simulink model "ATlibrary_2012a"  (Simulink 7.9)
settings: Solver=ode45  StartTime=0.0  StopTime=10.0  RelTol=1e-3
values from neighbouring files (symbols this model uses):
  params = []    [setParams.m]
  simopt = []    [setParams.m]
libraries: simulink x5, dspswit3 x1

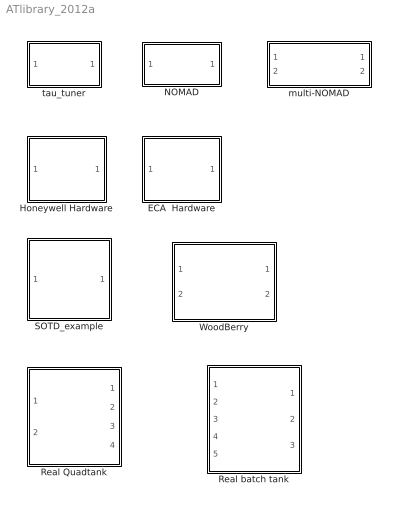
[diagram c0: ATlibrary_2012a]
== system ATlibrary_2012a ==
  ECA  Hardware : Subsystem
  Honeywell Hardware : Subsystem
  NOMAD : Subsystem  VariantObject=simopt.ID~=0
  Real Quadtank : Subsystem  AncestorBlock=tank/Real Quadtank  mask{h=0.01}
  Real batch tank : Subsystem  AncestorBlock=tank/Real Quadtank  mask{h=0.05}
  SOTD_example : Subsystem
  WoodBerry : Subsystem
  multi-NOMAD : Subsystem
  tau_tuner : Subsystem

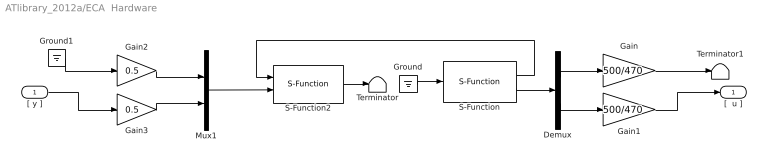
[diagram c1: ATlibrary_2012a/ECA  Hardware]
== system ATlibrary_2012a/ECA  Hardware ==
  "[ y ]" : Inport
  Demux : Demux  Outputs=2
  Gain : Gain  Gain=500/470
  Gain1 : Gain  Gain=500/470
  Gain2 : Gain  Gain=0.5
  Gain3 : Gain  Gain=0.5
  Ground : Ground
  Ground1 : Ground
  Mux1 : Mux  Inputs=2
  S-Function : S-Function  FunctionName=analogin  Parameters=simopt.h [1 0]  EnableBusSupport=off
  S-Function2 : S-Function  FunctionName=analogout  Parameters=simopt.h [1 0]  EnableBusSupport=off
  Terminator : Terminator
  Terminator1 : Terminator
  "[  u ]" : Outport  InitialOutput=0
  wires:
  Gain3/1 -> Mux1/2
  Gain2/1 -> Mux1/1
  Gain1/1 -> "[  u ]"/1
  Demux/2 -> Gain1/1
  Demux/1 -> Gain/1
  Gain/1 -> Terminator1/1
  Ground1/1 -> Gain2/1
  "[ y ]"/1 -> Gain3/1
  Mux1/1 -> S-Function2/2
  S-Function/2 -> Demux/1
  S-Function/1 -> S-Function2/1
  S-Function2/1 -> Terminator/1
  Ground/1 -> S-Function/1

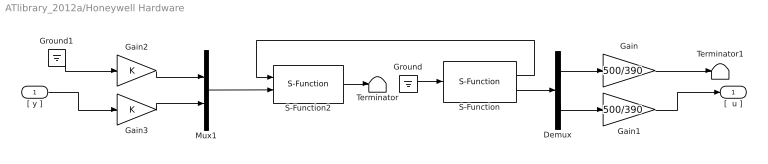
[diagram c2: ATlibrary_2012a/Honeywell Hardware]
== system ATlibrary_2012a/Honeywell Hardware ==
  "[ y ]" : Inport
  Demux : Demux  Outputs=2
  Gain : Gain  Gain=500/390
  Gain1 : Gain  Gain=500/390
  Gain2 : Gain
  Gain3 : Gain
  Ground : Ground
  Ground1 : Ground
  Mux1 : Mux  Inputs=2
  S-Function : S-Function  FunctionName=analogin  Parameters=simopt.h [1 0]  EnableBusSupport=off
  S-Function2 : S-Function  FunctionName=analogout  Parameters=simopt.h [1 0]  EnableBusSupport=off
  Terminator : Terminator
  Terminator1 : Terminator
  "[  u ]" : Outport  InitialOutput=0
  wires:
  Ground/1 -> S-Function/1
  S-Function2/1 -> Terminator/1
  S-Function/1 -> S-Function2/1
  S-Function/2 -> Demux/1
  Mux1/1 -> S-Function2/2
  "[ y ]"/1 -> Gain3/1
  Ground1/1 -> Gain2/1
  Gain/1 -> Terminator1/1
  Demux/1 -> Gain/1
  Demux/2 -> Gain1/1
  Gain1/1 -> "[  u ]"/1
  Gain2/1 -> Mux1/1
  Gain3/1 -> Mux1/2

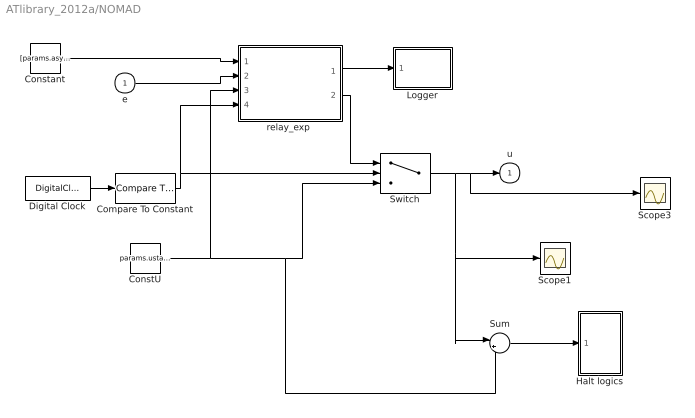
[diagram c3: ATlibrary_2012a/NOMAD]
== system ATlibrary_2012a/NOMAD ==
  e : Inport
  Compare To Constant : simulink/Logic and Bit Operations/Compare To Constant  relop=>=  const=params.expStartTime  OutDataTypeStr=boolean
  ConstU : Constant  Value=params.ustart  SampleTime=simopt.h
  Constant : Constant  Value=[params.asym simopt.h 1 simopt.uon params.hyst params.noiseMeasureTime]
  Digital Clock : DigitalClock  SampleTime=simopt.h
  Halt logics : Subsystem  VariantObject=Variant
  Logger : Subsystem
  Scope1 : Scope
  Scope3 : Scope
  Sum : Sum  Inputs=|+-
  Switch : Switch  Criteria=u2 ~= 0
  "relay_exp " : MATLAB Function  TreatAsAtomicUnit=on  SystemSampleTime=simopt.h  VariantObject=Variant
  u : Outport
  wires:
  Sum/1 -> Halt logics/1(u)
  Switch/1 -> Sum/1, Scope1/1, Scope3/1, u/1
  Compare To Constant/1 -> Switch/2, "relay_exp "/4(run_exp)
  ConstU/1 -> Sum/2, Switch/3, "relay_exp "/3(u0)
  Digital Clock/1 -> Compare To Constant/1
  "relay_exp "/1(result) -> Logger/1(result)
  Constant/1 -> "relay_exp "/1(relay_par)
  e/1 -> "relay_exp "/2(e)
  "relay_exp "/2(u) -> Switch/1

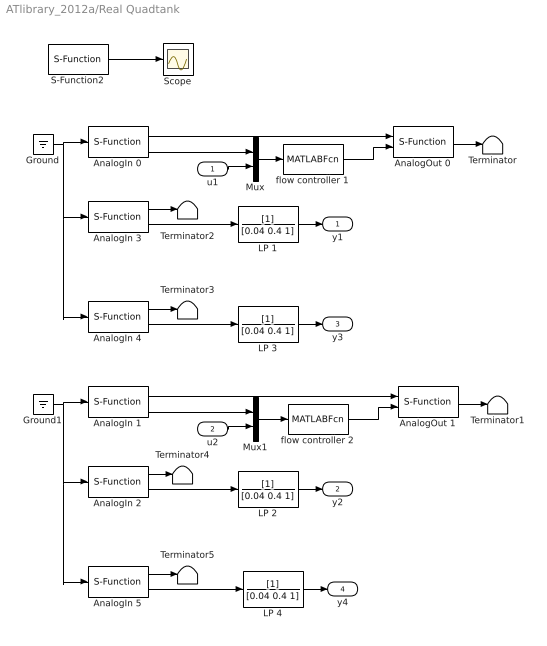
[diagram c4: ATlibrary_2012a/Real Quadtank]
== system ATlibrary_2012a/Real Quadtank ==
  u1 : Inport
  u2 : Inport  Port=2
  AnalogIn 0 : S-Function  FunctionName=analogin  Parameters=h [35]  EnableBusSupport=off
  AnalogIn 1 : S-Function  FunctionName=analogin  Parameters=h [34]  EnableBusSupport=off
  AnalogIn 2 : S-Function  FunctionName=analogin  Parameters=h [33]  EnableBusSupport=off
  AnalogIn 3 : S-Function  FunctionName=analogin  Parameters=h [31]  EnableBusSupport=off
  AnalogIn 4 : S-Function  FunctionName=analogin  Parameters=h [30]  EnableBusSupport=off
  AnalogIn 5 : S-Function  FunctionName=analogin  Parameters=h [32]  EnableBusSupport=off
  AnalogOut 0 : S-Function  FunctionName=analogout  Parameters=h [31]  EnableBusSupport=off
  AnalogOut 1 : S-Function  FunctionName=analogout  Parameters=h [30]  EnableBusSupport=off
  Ground : Ground
  Ground1 : Ground
  LP {1..4} (4 alike) : TransferFcn  Denominator=[0.04 0.4 1]
  Mux : Mux  Inputs=2
  Mux1 : Mux  Inputs=2
  S-Function2 : S-Function  FunctionName=realtimer  Parameters=h  EnableBusSupport=off
  Scope : Scope
  Terminator{,1..5} (6 alike) : Terminator
  flow controller 1 : MATLABFcn  MATLABFcn=flowCtrl1  SampleTime=0.01
  flow controller 2 : MATLABFcn  MATLABFcn=flowCtrl2  SampleTime=0.01
  y1 : Outport
  y2 : Outport  Port=2
  y3 : Outport  Port=3
  y4 : Outport  Port=4
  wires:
  S-Function2/1 -> Scope/1
  AnalogIn 0/1 -> AnalogOut 0/1
  AnalogOut 0/1 -> Terminator/1
  AnalogIn 1/1 -> AnalogOut 1/1
  AnalogOut 1/1 -> Terminator1/1
  AnalogIn 3/2 -> LP 1/1
  AnalogIn 4/2 -> LP 3/1
  Ground/1 -> AnalogIn 0/1, AnalogIn 3/1, AnalogIn 4/1
  AnalogIn 3/1 -> Terminator2/1
  AnalogIn 4/1 -> Terminator3/1
  AnalogIn 2/2 -> LP 2/1
  AnalogIn 5/2 -> LP 4/1
  Ground1/1 -> AnalogIn 5/1, AnalogIn 2/1, AnalogIn 1/1
  AnalogIn 2/1 -> Terminator4/1
  AnalogIn 5/1 -> Terminator5/1
  u1/1 -> Mux/2
  Mux/1 -> flow controller 1/1
  flow controller 1/1 -> AnalogOut 0/2
  u2/1 -> Mux1/2
  Mux1/1 -> flow controller 2/1
  flow controller 2/1 -> AnalogOut 1/2
  AnalogIn 1/2 -> Mux1/1
  AnalogIn 0/2 -> Mux/1
  LP 1/1 -> y1/1
  LP 3/1 -> y3/1
  LP 2/1 -> y2/1
  LP 4/1 -> y4/1

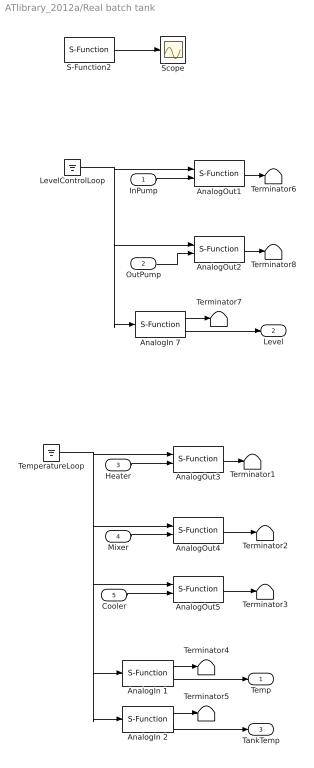
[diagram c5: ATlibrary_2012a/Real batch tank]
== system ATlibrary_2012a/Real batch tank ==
  InPump : Inport
  OutPump : Inport  Port=2
  Heater : Inport  Port=3
  Mixer : Inport  Port=4
  Cooler : Inport  Port=5
  AnalogIn 1 : S-Function  FunctionName=analogin  Parameters=h [30]  EnableBusSupport=off
  AnalogIn 2 : S-Function  FunctionName=analogin  Parameters=h [37]  EnableBusSupport=off
  AnalogIn 7 : S-Function  FunctionName=analogin  Parameters=h [31]  EnableBusSupport=off
  AnalogOut1 : S-Function  FunctionName=analogout  Parameters=h [32]  EnableBusSupport=off
  AnalogOut2 : S-Function  FunctionName=analogout  Parameters=h [33]  EnableBusSupport=off
  AnalogOut3 : S-Function  FunctionName=analogout  Parameters=h [30]  EnableBusSupport=off
  AnalogOut4 : S-Function  FunctionName=analogout  Parameters=h [34]  EnableBusSupport=off
  AnalogOut5 : S-Function  FunctionName=analogout  Parameters=h [31]  EnableBusSupport=off
  LevelControlLoop : Ground
  S-Function2 : S-Function  FunctionName=realtimer  Parameters=h  EnableBusSupport=off
  Scope : Scope
  TemperatureLoop : Ground
  Terminator{1..8} (8 alike) : Terminator
  Temp : Outport
  Level : Outport  Port=2
  TankTemp : Outport  Port=3
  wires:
  S-Function2/1 -> Scope/1
  AnalogIn 7/1 -> Terminator7/1
  LevelControlLoop/1 -> AnalogIn 7/1, AnalogOut2/1, AnalogOut1/1
  AnalogIn 7/2 -> Level/1
  AnalogOut1/1 -> Terminator6/1
  OutPump/1 -> AnalogOut2/2
  AnalogOut2/1 -> Terminator8/1
  InPump/1 -> AnalogOut1/2
  TemperatureLoop/1 -> AnalogOut4/1, AnalogOut5/1, AnalogIn 1/1, AnalogIn 2/1, AnalogOut3/1
  AnalogOut3/1 -> Terminator1/1
  Heater/1 -> AnalogOut3/2
  AnalogOut4/1 -> Terminator2/1
  Mixer/1 -> AnalogOut4/2
  AnalogOut5/1 -> Terminator3/1
  Cooler/1 -> AnalogOut5/2
  AnalogIn 1/1 -> Terminator4/1
  AnalogIn 1/2 -> Temp/1
  AnalogIn 2/1 -> Terminator5/1
  AnalogIn 2/2 -> TankTemp/1

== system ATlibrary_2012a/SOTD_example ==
  u : Inport  SampleTime=simopt.h
  Transfer Fcn : TransferFcn  Denominator=[1 4 6 4 1]
  y : Outport  SampleTime=simopt.h
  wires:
  Transfer Fcn/1 -> y/1
  u/1 -> Transfer Fcn/1

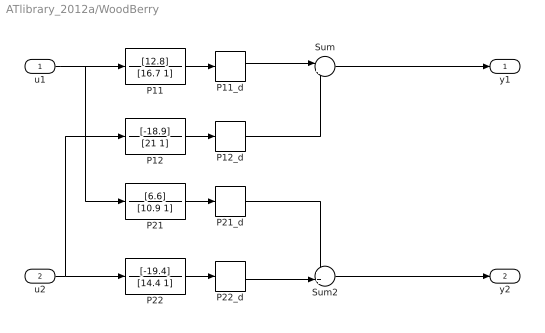
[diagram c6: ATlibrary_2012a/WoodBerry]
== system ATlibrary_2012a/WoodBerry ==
  u1 : Inport
  u2 : Inport  Port=2
  P11 : TransferFcn  Numerator=[12.8]  Denominator=[16.7 1]
  P11_d : TransportDelay
  P12 : TransferFcn  Numerator=[-18.9]  Denominator=[21 1]
  P12_d : TransportDelay  DelayTime=3
  P21 : TransferFcn  Numerator=[6.6]  Denominator=[10.9 1]
  P21_d : TransportDelay  DelayTime=7
  P22 : TransferFcn  Numerator=[-19.4]  Denominator=[14.4 1]
  P22_d : TransportDelay  DelayTime=3
  Sum : Sum  Inputs=|++
  Sum2 : Sum  Inputs=++|
  y1 : Outport
  y2 : Outport  Port=2
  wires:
  P11/1 -> P11_d/1
  P11_d/1 -> Sum/1
  Sum/1 -> y1/1
  u1/1 -> P11/1, P21/1
  P12/1 -> P12_d/1
  P12_d/1 -> Sum/2
  u2/1 -> P12/1, P22/1
  P21/1 -> P21_d/1
  P21_d/1 -> Sum2/1
  P22/1 -> P22_d/1
  P22_d/1 -> Sum2/2
  Sum2/1 -> y2/1

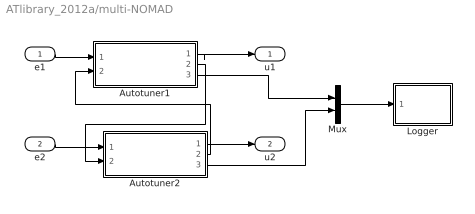
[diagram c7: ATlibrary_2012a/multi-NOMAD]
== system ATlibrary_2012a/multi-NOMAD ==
  e1 : Inport
  e2 : Inport  Port=2
  Autotuner1 : Subsystem
  Autotuner2 : Subsystem
  Logger : Subsystem
  Mux : Mux  Inputs=2
  u1 : Outport
  u2 : Outport  Port=2
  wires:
  Autotuner1/2(done) -> Autotuner2/2(other_done)
  Autotuner2/2(done) -> Autotuner1/2(other_done)
  Autotuner1/1(u) -> u1/1
  Autotuner2/1(u) -> u2/1
  e1/1 -> Autotuner1/1(e)
  e2/1 -> Autotuner2/1(e)
  Autotuner1/3(result1) -> Mux/1
  Autotuner2/3(result2) -> Mux/2
  Mux/1 -> Logger/1(result)

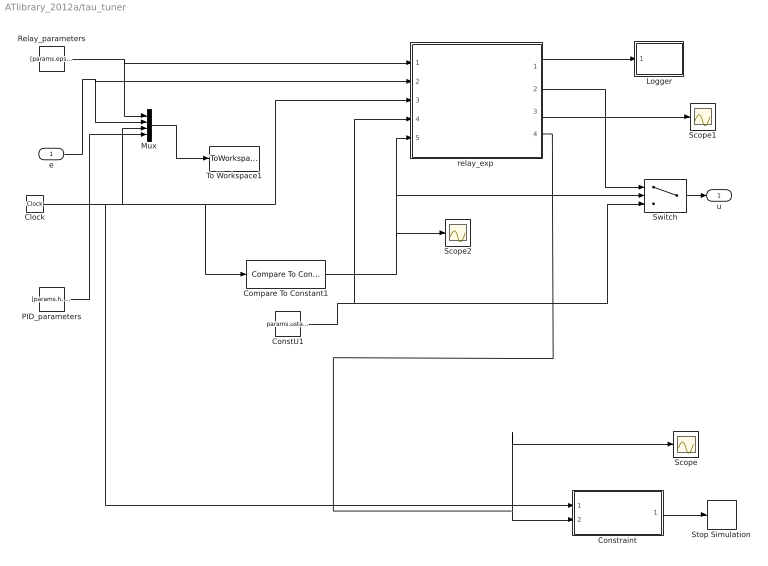
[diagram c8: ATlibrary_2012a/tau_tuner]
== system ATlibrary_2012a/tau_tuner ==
  e : Inport  SampleTime=simopt.h
  Clock : Clock
  Compare To Constant1 : simulink/Logic and Bit Operations/Compare To Constant  relop=>=  const=params.expStartTime  OutDataTypeStr=boolean
  ConstU1 : Constant  Value=params.ustart  SampleTime=simopt.h
  Constraint : MATLAB Function  TreatAsAtomicUnit=on
  Logger : Subsystem
  Mux : Mux
  PID_parameters : Constant  Value=[params.h, params.equi]  SampleTime=simopt.h
  Relay_parameters : Constant  Value=[params.eps, params.asym, params.h, 2,12,1, params.uon,params.hyst,params.noiseMeasureTime, 0]  SampleTime=simopt.h
  Scope : Scope
  Scope1 : Scope
  Scope2 : Scope
  Stop Simulation : Stop
  Switch : Switch  Criteria=u2 ~= 0
  To Workspace1 : ToWorkspace  VariableName=result1  SampleTime=-1  SaveFormat=Timeseries
  "relay_exp " : MATLAB Function  TreatAsAtomicUnit=on
  u : Outport  SampleTime=simopt.h
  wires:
  Mux/1 -> To Workspace1/1
  Switch/1 -> u/1
  e/1 -> "relay_exp "/2(e), Mux/2
  Relay_parameters/1 -> "relay_exp "/1(relay_par), Mux/1
  PID_parameters/1 -> Mux/4
  "relay_exp "/2(u) -> Switch/1
  Compare To Constant1/1 -> Scope2/1, "relay_exp "/5(run_exp), Switch/2
  ConstU1/1 -> "relay_exp "/4(u_ref), Switch/3
  "relay_exp "/4(done) -> Constraint/2(done), Scope/1
  Clock/1 -> Compare To Constant1/1, "relay_exp "/3(t), Mux/3, Constraint/1(time)
  "relay_exp "/3(PID_param) -> Scope1/1
  "relay_exp "/1(result) -> Logger/1(result)
  Constraint/1(stop) -> Stop Simulation/1

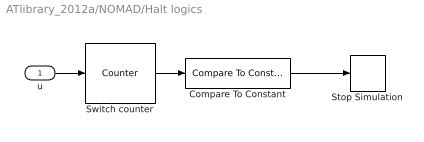
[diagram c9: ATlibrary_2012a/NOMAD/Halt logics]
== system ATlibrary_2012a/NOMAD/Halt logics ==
  u : Inport
  Compare To Constant : simulink/Logic and Bit Operations/Compare To Constant  relop=>=  const=params.switches  OutDataTypeStr=boolean
  Stop Simulation : Stop
  Switch counter : dspswit3/Counter  Direction=Up  CountEvent=Either edge  CounterSize=User defined  MaxCount=params.switches  InitialCount=0  Output=Count  HitValue=32  ResetInput=off  SamplesPerFrame=1  Ts=1  CntDtype=double  HitDtype=Logical
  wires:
  Compare To Constant/1 -> Stop Simulation/1
  u/1 -> Switch counter/1
  Switch counter/1 -> Compare To Constant/1

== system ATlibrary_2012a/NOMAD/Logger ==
  result : Inport  SampleTime=simopt.h
  Logger : ToWorkspace  VariableName=result  SampleTime=simopt.h  SaveFormat=Structure With Time
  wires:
  result/1 -> Logger/1

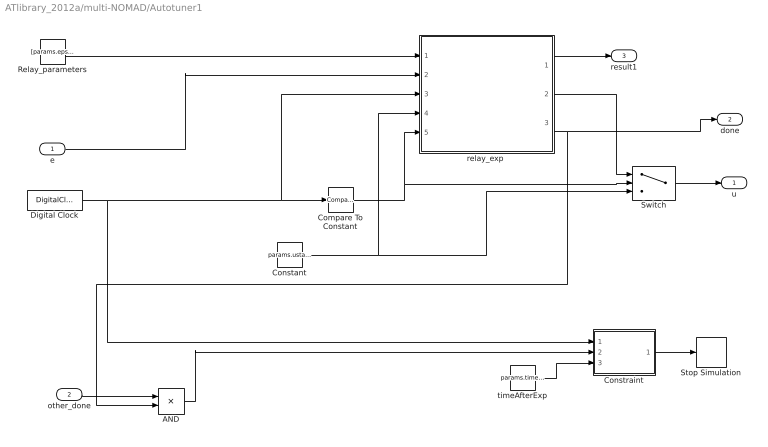
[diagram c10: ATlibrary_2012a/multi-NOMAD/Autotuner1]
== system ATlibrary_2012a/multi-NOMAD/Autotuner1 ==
  e : Inport
  other_done : Inport  Port=2
  AND : Product
  Compare To Constant : simulink/Logic and Bit Operations/Compare To Constant  relop=>=  const=params.expStartTime  OutDataTypeStr=boolean
  Constant : Constant  Value=params.ustart  SampleTime=simopt.h
  Constraint : MATLAB Function  TreatAsAtomicUnit=on  SystemSampleTime=simopt.h
  Digital Clock : DigitalClock  SampleTime=simopt.h
  Relay_parameters : Constant  Value=[params.eps, params.gamma, simopt.h, params.low_limit, params.dev_limit, 1 , params.uon, params.hyst, params.noiseMeasureTime, 1, params.gamma2, params.switches, params.ystep, params.ustep]  SampleTime=simopt.h
  Stop Simulation : Stop
  Switch : Switch  Criteria=u2 ~= 0
  "relay_exp " : MATLAB Function  TreatAsAtomicUnit=on  SystemSampleTime=simopt.h
  timeAfterExp : Constant  Value=params.timeAfterExp
  u : Outport
  done : Outport  Port=2
  result1 : Outport  Port=3
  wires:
  Switch/1 -> u/1
  Relay_parameters/1 -> "relay_exp "/1(relay_par)
  "relay_exp "/2(u) -> Switch/1
  Compare To Constant/1 -> Switch/2, "relay_exp "/5(run_exp)
  Constant/1 -> "relay_exp "/4(u_ref), Switch/3
  e/1 -> "relay_exp "/2(e)
  Digital Clock/1 -> "relay_exp "/3(t), Compare To Constant/1, Constraint/1(time)
  Constraint/1(stop) -> Stop Simulation/1
  AND/1 -> Constraint/2(all_done)
  other_done/1 -> AND/1
  "relay_exp "/3(done) -> AND/2, done/1
  timeAfterExp/1 -> Constraint/3(timeAfterExp)
  "relay_exp "/1(result) -> result1/1

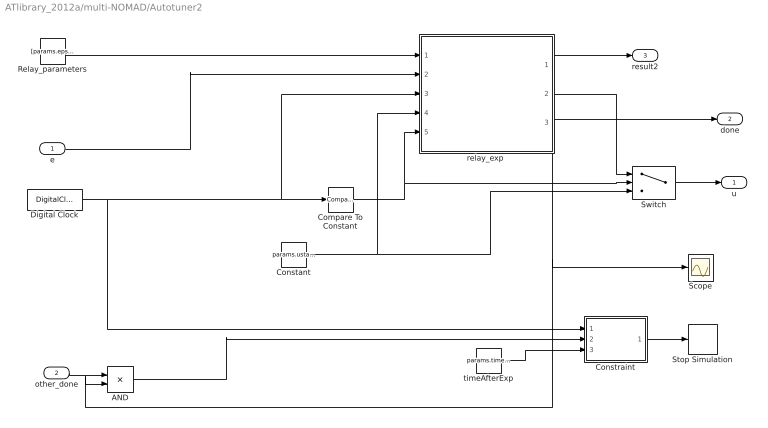
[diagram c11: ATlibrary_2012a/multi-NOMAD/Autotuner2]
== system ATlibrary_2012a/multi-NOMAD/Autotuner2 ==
  e : Inport
  other_done : Inport  Port=2
  AND : Product
  Compare To Constant : simulink/Logic and Bit Operations/Compare To Constant  relop=>=  const=params.expStartTime  OutDataTypeStr=boolean
  Constant : Constant  Value=params.ustart  SampleTime=simopt.h
  Constraint : MATLAB Function  TreatAsAtomicUnit=on  SystemSampleTime=simopt.h
  Digital Clock : DigitalClock  SampleTime=simopt.h
  Relay_parameters : Constant  Value=[params.eps,params.gamma, simopt.h,params.low_limit,params.dev_limit,1,params.uon,params.hyst,params.noiseMeasureTime,1,params.gamma2,params.switches,params.ystep,params.ustep]  SampleTime=simopt.h
  Scope : Scope
  Stop Simulation : Stop
  Switch : Switch  Criteria=u2 ~= 0
  "relay_exp " : MATLAB Function  TreatAsAtomicUnit=on  SystemSampleTime=simopt.h
  timeAfterExp : Constant  Value=params.timeAfterExp
  u : Outport
  done : Outport  Port=2
  result2 : Outport  Port=3
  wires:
  Switch/1 -> u/1
  Relay_parameters/1 -> "relay_exp "/1(relay_par)
  "relay_exp "/2(u) -> Switch/1
  e/1 -> "relay_exp "/2(e)
  "relay_exp "/1(result) -> result2/1
  Constraint/1(stop) -> Stop Simulation/1
  AND/1 -> Constraint/2(all_done)
  other_done/1 -> AND/1
  "relay_exp "/3(done) -> Scope/1, AND/2, done/1
  timeAfterExp/1 -> Constraint/3(timeAfterExp)
  Compare To Constant/1 -> Switch/2, "relay_exp "/5(run_exp)
  Constant/1 -> "relay_exp "/4(u_ref), Switch/3
  Digital Clock/1 -> "relay_exp "/3(t), Compare To Constant/1, Constraint/1(time)

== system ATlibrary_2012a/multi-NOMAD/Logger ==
  result : Inport  SampleTime=simopt.h
  Logger : ToWorkspace  VariableName=result  SampleTime=simopt.h  SaveFormat=Structure With Time
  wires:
  result/1 -> Logger/1

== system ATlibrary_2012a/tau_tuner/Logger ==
  result : Inport  SampleTime=simopt.h
  Logger : ToWorkspace  VariableName=result  SampleTime=simopt.h  SaveFormat=Structure With Time
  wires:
  result/1 -> Logger/1

== matlab function NOMAD/relay_exp
 ==
function [result, u] = relay_function(relay_par, e, u0, run_exp)

%%%%%%%%%% Definitions and default values %%%%%%%%%%%%%%
y=-e;
% Relay parameters, values from workspace.
persistent d1 d2 u_on u_off h
gamma = relay_par(1);
t_sample = relay_par(2);
bigYup = relay_par(3);
relayMaxDev = relay_par(4);
def_h = relay_par(5);
noiseMeasureTime = relay_par(6);

persistent yref uref
if isempty(d2)
    h=def_h;
    % These values are re-assigned later in the program so they won't be
    % used. But they are assigned in an if-statement so the program doesn't
    % understand that they will always be assigned before they are used.
    d1 = gamma;
    d2 = 1;
    u_on =  d1;
    u_off = -d2;
    uref = u0;
    yref = 0;
end

persistent u_old startup Ksign
if isempty(u_old)
    u_old = uref;
    Ksign = 1; % Will be re-assigned during the startup phase
end

persistent sample
if isempty(sample)
    sample = 0;
end


%%%%%%%%% Startup  params %%%%%%%%%%%
persistent a b c tff exp_t yh yl measureNoise first
if isempty(startup)
    tff = 1/t_sample; % Usually 5 but to not make the startup phase a too large part of the id data in the ETFA paper we decreased it! Want the ramp-up to be a certain time, according to Tore about 3-5s 
    b = 40;
    c = relayMaxDev/(b-1);
    a = uref-c;
    measureNoise = 1;
    startup = 0;
    yh = 0;
    yl = 0;
    first = true;
end
%%%%%%%%%%%%%%%%%%%%%%%%%%%%%%%%%%%%%%%%%%%%%%

if run_exp == 0
    u = 0;
    result = [0 0 0];
    return
end


%%%%%%%%%%%%% Program running %%%%%%%%%%%%%%%%%

sample = sample+1;
if sample > 1
end

% %%%%%%%%% Startup %%%%%%%%%%%%
 if measureNoise == 1
    if first 
        uref = u0;
        yref = y;
        first = false;
        yh = yref;
        yl = yref;
    end
    u = uref;
    if sample < noiseMeasureTime/t_sample
        yh = max(yh,y);
        yl = min(yl,y);
    else
        noise = (yh-yl)/2;
        yref = (yh+yl)/2;
        h = max(2*noise, def_h);
        measureNoise = 0;
        startup = 1;
    end
 elseif startup == 1
    exp_t = sample-noiseMeasureTime/t_sample;
    a = uref-c;
        u = (a+c*b^(exp_t/tff));
        if abs(u) > relayMaxDev+uref
            u = (relayMaxDev+uref);
        end
        if exp_t > 1
            ydev = y-yref; 
            if abs(ydev) > h % reached outside hysteresis, stop and decide Ksign
                Ksign = ydev/abs(ydev)
                if bigYup == 1
                    %d1 = min(relayMaxDev, gamma*abs(u-uref));
                    d1 = min(relayMaxDev, abs(u-uref)); %could be a problem to have the large/small this way but prefer it. 
                    d2 = d1/gamma;
                else
                    %d2 = min(relayMaxDev, gamma*abs(u-uref));
                    d2 = min(relayMaxDev, abs(u-uref));
                    d1 = d2/gamma;
                end
                startup = 0;
                u_on = uref+Ksign*d1;
                u_off = uref-Ksign*d2;
                if Ksign > 0
                    u = u_off;
                else
                    u = u_on;
                end
            elseif exp_t > tff
                u = uref+relayMaxDev;
            end
        end
 else
    %%%%%% Update amplitudes %%%%%%%
    u_on = uref+Ksign*d1;
    u_off = uref-Ksign*d2;
    %%%%%% Calculate new u %%%%%%%%%
    if y <= yref-h
        u = u_on;
    elseif y < yref+h && y > yref-h
        u = u_old;
    else u = u_off;
    end
 end
%%%% store data %%%%%%
u_old = u;
result = [yref, uref, h];

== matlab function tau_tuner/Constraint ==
%function stop = Constraint(tstop, time, done)
function stop = Constraint(time, done)
%#codegen
persistent tstopp
if isempty(tstopp)
    tstopp = 10000;
end
if done == 1
    tstopp = time;
end
if time > tstopp; %+params.timeAfterExp;
    stop = 1;
else
    stop = 0;
end

== matlab function tau_tuner/relay_exp
 ==
function [result, u, PID_param, done]= relay_exp(relay_par, e,t, u_ref, run_exp)


%%%%%%%%%% Definitions and default values %%%%%%%%%%%%%%
y = -e;
% Relay parameters, values from workspace.
persistent d1 d2 u_on u_off h
epsilon = relay_par(1);
gamma = relay_par(2); 
t_sample = relay_par(3);
low_limit_f = relay_par(4);
upp_limit_f = relay_par(5);
bigYup = relay_par(6);
relayMaxDev = relay_par(7);
def_h = relay_par(8);
noiseMeasureTime = relay_par(9);
fixAmp = relay_par(10);

persistent yref uref resultvec
if isempty(d2)
    h=def_h;
    % These values are assigned to their values later in the code, but in an if-statement
    % so the program doesn't understand that they will always be assigned. 
    d1 = gamma;
    d2 = 1;
    u_on =  d1;
    u_off = -d2;
    uref = 0;
    yref = y;
    resultvec = zeros(22,1);
end

% Creating arrays for data logging
maxlength = 1000000;
persistent uvec yvec tvec 
if isempty(uvec)
    uvec = zeros(1,maxlength);
    yvec = zeros(1,maxlength);
    tvec = zeros(1,maxlength);
end

persistent sample
if isempty(sample)
    sample = 0;
end

persistent startup Ksign startup_switch amp_changed
if isempty(Ksign)
    Ksign = 1; % Is found and assigned during the startup phase
    startup_switch = 0; 
    amp_changed = 0;
end

persistent param 
if isempty(param)
    param = [1, 10, 0]; % Should be an input somehow if an existing PID controller is used first
end
PID_param = param; % Not allowed to have a persistent variable as output so had to do like this
done = 0;
finished = false;

% To handle switches
persistent switching_times switch_index last_switch_sample
if isempty(switching_times)
    switching_times = zeros(1,100); % Larger than necessary
    switch_index = 1;
    last_switch_sample = 1;
end

%%%%%%%%% Startup  params %%%%%%%%%%%
persistent a b c ttf exp_t yh yl measureNoise first
if isempty(startup)
    uvec(1) = uref;
    yvec(1) = yref;
    tvec(1) = 0;
    ttf = 5/t_sample; % Want to run the exponential growth for a certain time, not a number of samples. According to Tore about 3-5s 
    b = 40;
    c = relayMaxDev/(b-1);
    a = uvec(1)-c;
    measureNoise = 1;
    startup = 0;
    yh = 0;
    yl = 0;
    first = true;
end
%%%%%%%%%%%%%%%%%%%%%%%%%%%%%%%%%%%%%%%%%%%%%%%

result = resultvec;
if run_exp == 0
    done = 0;
    u = 0;
    PID_param = param;
    return
end
if fixAmp == 1
   d1 = upp_limit_f;
   d2 = low_limit_f;
end
%%%%%%%%%%%%% Program running %%%%%%%%%%%%%%%%%
sample = sample+1;
if sample > 1
  yvec(sample-1) = y; % store inputs
  tvec(sample) = t;
end

%%%%%%%%% Startup %%%%%%%%%%%%
if measureNoise == 1
    if first 
        uref = u_ref;
        yref = y;
        first = false;
        yh = yref;
        yl = yref;
    end
    u = uref;
    if sample < noiseMeasureTime/t_sample
        yh = max(yh,y);
        yl = min(yl,y);
    else
        resultvec(13) = yh;
        resultvec(14) = yl;
        noise = (yh-yl)/2;
        yref = (yh+yl)/2;
        resultvec(15) = yref;
        resultvec(16) = uref;
        h = max(2*noise, def_h);
        resultvec(12) = h;
        measureNoise = 0;
        startup = 1;
    end
elseif startup == 1
    exp_t = sample-noiseMeasureTime/t_sample; % this should be zero the first sample
    a = uref-c;
        u = a+c*b^(exp_t/ttf);
        if u > relayMaxDev+uref
            u = relayMaxDev+uref;
        end
        if exp_t > 1
            ydev = y-yref; 
            if abs(ydev) > h % when reached outside hysteresis, stop and decide Ksign
                Ksign = ydev/abs(ydev)
                if bigYup == 1
                    d1 = min(relayMaxDev, gamma*abs(u-uref));
                    d2 = d1/gamma;
                else
                    d2 = min(relayMaxDev, gamma*abs(u-uref));
                    d1 = d2/gamma;
                end
                startup = 0;
                startup_switch = 1; % To not immediately change the new amplitude.
            elseif exp_t > ttf
                u = uref+relayMaxDev;
            end
        end
elseif done == 0
    %%%%%% Update amplitudes %%%%%%%
    u_on = uref+Ksign*d1;
    u_off = uref-Ksign*d2;
    %%%%%% Calculate new u %%%%%%%%%
    u = rel_func(y,uvec(sample-1),u_on, u_off,yref,h);
else 
    u = 0; % If the experiment aren't running no control signal should be calculated here
    % This script shouldn't be running in those cases but somehow it seems
    % to do.
end
%%%% store data %%%%%%
uvec(sample) = u;

%%%%%%% At switching points %%%%%%%
if sample>1 && (uvec(sample)-uref)*(uvec(sample-1)-uref) < 0
    switching_times(switch_index) = tvec(sample);
    low_limit = low_limit_f*h;
    upp_limit = upp_limit_f*h;
    ratio = check_amplitudes(yvec(last_switch_sample:sample-1)-yref, upp_limit, low_limit, gamma);
    if fixAmp == 1
        ratio = 1;
    end
    if amp_changed == 1 % To not change two consecutive half periods...
        ratio = 1;
        amp_changed = 0;
    end
    if (ratio > 1.01 || ratio < 0.99) && startup_switch ~= 1 
        if max(d1,d2)*ratio > relayMaxDev
            if max(d1,d2) == relayMaxDev
                ratio_forced = 1
                %ratio = 1;
            else
                ratio = relayMaxDev/max(d1,d2);
                d1 = d1*ratio;
                d2 = d2*ratio;
                switch_index = 0; % to reset convergence checks if changed amplitude.
                amp_changed = 1;
            end
            
       else
            d1 = d1*ratio;
            d2 = d2*ratio;
            switch_index = 0; % To reset convergence checks if changed amplitude.
            amp_changed = 1;
       end
       if uvec(sample) == u_on
           u = uref+Ksign*d1;
       elseif uvec(sample) == u_off
           u = uref-Ksign*d2;
       else
           error = 1
       end
       uvec(sample) = u;
    end
    startup_switch = 0;
    if switch_index > 3
        tp = switching_times(switch_index)-switching_times(switch_index-2);
        tp_old = switching_times(switch_index-1)-switching_times(switch_index-3);
        resultvec(19) = tp;
        resultvec(20) = tp_old;
        if abs(tp-tp_old)<tp_old*epsilon
            finished = true;
            tstop = tvec(sample);
            resultvec(17) = tstop;
        end
    end
    last_switch_sample = sample;
    switch_index = switch_index+1;
end


% Checks if converged, in that case collect info and call a method that
% calculates a model and PI/PID parameters
if finished == true
    tsim = tvec(1:sample);
    usim = uvec(1:sample)-uref;
    ysim = yvec(1:sample)-yref;
        u1 = usim(1:end-1);
        u2 = usim(2:end);
        switches = find(u1.*u2<0);
        yp = ysim(switches(end-2):switches(end));
        up = usim(switches(end-2):switches(end));
        tp = tsim(switches(end-2):switches(end));
        y_int = trapz(tp,yp);
        u_int = trapz(tp,up);
        resultvec(21) = y_int;
        resultvec(22) = u_int;
    [ton toff] = calc_ton_toff(usim, switching_times(1:switch_index-1), u_on-uref);
    resultvec(8) = ton;
    resultvec(9) = toff;
    %%%%% Calulating tau %%%%%
    rho = max(ton, toff)/min(ton, toff);
    tau = min(1, max((gamma-rho)/((gamma-1)*(0.35*rho+0.65)),0)) %Min&max if something strange would occur.
    resultvec(1) = tau;
  
    if tau > 0.1 % this condition needs to be considered more closely
        [K,T,L] = calc_FOTD_params(u_int,y_int,d1,d2,h,ton,toff,tau);
        if tau > 0.6
           [Kc, Ti, Td] = calc_AMIGO_PI(K,T,L);
        else
            [Kc, Ti, Td] = calc_AMIGO_PID(K,T,L);
        end
        resultvec(2) = K;
        resultvec(3) = T;
        resultvec(4) = L;
        resultvec(5) = Kc;
        resultvec(6) = Ti;
        resultvec(7) = Td;
    else
        [kv, L] = calc_integrating_params(y_int, u_on-uref, u_off-uref, ton, toff, h);
        %[Kc, Ti, Td] = calc_AMIGO_int_PI(kv, L);
        [Kc, Ti, Td] = calc_AMIGO_int_PID(kv, L); % Which one do I want?
        resultvec(2) = kv;
        resultvec(3) = -1;
        resultvec(4) = L;
        resultvec(5) = Kc;
        resultvec(6) = Ti;
        resultvec(7) = Td;
    end
    done = 1;
    param = [Kc, Ti, Td];
    resultvec(10) = d1;
    resultvec(11) = d2;
    resultvec(18) = done;
    resultvec
end
end


% ---------------------------------
 function ratio = check_amplitudes(y, upper_limit, lower_limit, gamma)
        % Is checked at every switching point and sends in y = y_vec-yref
        % for the entire half period. No point to check at other time
        % instances!
        ratio1 = max(abs(y))/upper_limit; % Top value deviates too much if > 1
        ratio2 = max(abs(y))/lower_limit; % Top value too close to hysteresis limit if < 1.
     
        if ratio1 > 1
            ratio = (upper_limit+lower_limit*gamma)/(2*max(abs(y))); 
        elseif ratio2 < 1
            ratio = (lower_limit+upper_limit/gamma)/(2*max(abs(y)));
        else
            ratio =1;
        end
    end
%---------------------------------------

function u = rel_func(y,uold,uon,uoff,yref,h)
  if y <= yref-h
    u = uon;
  elseif y < yref+h && y > yref-h
    u = uold;
  else u = uoff;
  end
end

% --------------------------------
function [ton, toff] = calc_ton_toff(u, switching_times, u_on)

if u(end-1) == u_on
    ton = switching_times(end)-switching_times(end-1);
    toff = switching_times(end-1)-switching_times(end-2);
else
    toff = switching_times(end)-switching_times(end-1);
    ton = switching_times(end-1)-switching_times(end-2);
end
end

% ---------------------------------------------------

function [kstart tstart lstart] = calc_FOTD_params(u_int,y_int,d1,d2,h, ton, toff, tau)
kstart=y_int/u_int;
LdivT = tau/(1-tau);
% Equations from commit 2015-02-10
u_int
y_int
d1
d2
h
ton
toff
tau
tstart1 = ton/log((h/abs(kstart)-d2+exp(LdivT)*(d1+d2))/(d1-h/abs(kstart)));
tstart2 = toff/log((h/abs(kstart)-d1+exp(LdivT)*(d1+d2))/(d2-h/abs(kstart)));
tstart = (tstart1+tstart2)/2;
lstart = tstart*LdivT;
end

% --------------------------------------------

function [K, Ti, Td] = calc_AMIGO_PI(Kp,T,L)
K = 0.15/Kp+(0.35-L*T/(L+T)^2)*T/(Kp*L);
Ti = 0.35*L+13*L*T^2/(T^2+12*L*T+7*L^2);
Td = 0;
end

function [K, Ti, Td] = calc_AMIGO_PID(Kp,T,L)
K = (0.2*L+0.45*T)/(Kp*L);
Ti = (0.4*L+0.8*T)/(L+0.1*T)*L;
Td = 0.5*L*T/(0.3*L+T);
end

% --------------------------------------------
function [kv, L] = calc_integrating_params(y_int, uon, uoff, ton, toff, h)
%Equations from commit 2015-02-10
y_int
uon
uoff
ton
toff
h

kv = 2*y_int/(ton*toff*(uon+uoff))+2*h/(uon*ton);
L = (uon*ton-2*h/kv)/(uon-uoff);
if L < 0
    L = 1e-3;
end
end

% -------------------------------------------
function [K, Ti, Td] = calc_AMIGO_int_PI(Kv, L)
K = 0.35/(Kv*L);
Ti = 13.4*L;
Td = 0;
end

function [K, Ti, Td] = calc_AMIGO_int_PID(Kv, L)
K = 0.45/(Kv*L);
Ti = 8*L;
Td = 0.5*L;
end

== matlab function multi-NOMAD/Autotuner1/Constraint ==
%function stop = Constraint(tstop, time, done)
function stop = Constraint(time, all_done, timeAfterExp)
%#codegen
persistent tstopp first
if isempty(tstopp)
    tstopp = 10000;
    first = true;
end
if all_done == 1 && first 
    tstopp = time;
    first = false;
end
if time > tstopp+timeAfterExp;
    stop = 1;
else
    stop = 0;
end

== matlab function multi-NOMAD/Autotuner1/relay_exp
 ==
function [result, u, done]= relay_exp(relay_par, e,t, u_ref, run_exp)


%%%%%%%%%% Definitions and default values %%%%%%%%%%%%%%
y = -e;
% Relay parameters, values from workspace.
persistent d1 d2 u_on u_off h
gamma = relay_par(11); % index 2 is gamma, 11 is gamma2 
t_sample = relay_par(3);
bigYup = relay_par(6);
relayMaxDev = relay_par(7);
def_h = relay_par(8);
noiseMeasureTime = relay_par(9);
maxSwitches = relay_par(12);
ystep = relay_par(13);
ustep = relay_par(14);

persistent yref uref
if isempty(d2)
    h=def_h; % these values will be re-assigned later and never used.
    d1 = gamma;
    d2 = 1;
    u_on =  d1;
    u_off = -d2;
    uref = 0;
    yref = 0;
end

persistent u_old resultvec
if isempty(u_old)
    u_old = uref;
    resultvec = zeros(23,1);
end

persistent sample
if isempty(sample)
    sample = 0;
end

persistent startup Ksign
if isempty(Ksign)
    Ksign = 1; % Is re-assigned during at the startup phase
end

persistent param done_per
if isempty(param)
    param = [1.1, 16, 0]; % Quadtank minfas (should be an input somehow if existing PID parameters are used to bring it to its working point)
    done_per = 0;
end
PID_param = param;
done = done_per;

% To handle switches
persistent switching_times switch_index 
if isempty(switching_times)
    switching_times = zeros(1,20); % Shouldn't need to be so large
    switch_index = 1;
end

%%%%%%%%% Startup  params %%%%%%%%%%%
persistent a b c tff exp_t yh yl measureNoise first
if isempty(startup)
    tff = 5/t_sample; % According to Tore about 3-5s is appropriate for the startup growth 
    b = 40;
    c = relayMaxDev/(b-1);
    a = uref-c;
    measureNoise = 1;
    startup = 0;
    yh = 0;
    yl = 0;
    first = true;
end
%%%%%%%%%%%%%%%%%%%%%%%%%%%%%%%%%%%%%%%%%%%%%%%

result = resultvec;
if run_exp == 0
    u = 0;
    PID_param = param;
    return
end

%%%%%%%%%%%%% Program running %%%%%%%%%%%%%%%%%
sample = sample+1;

%%%%%%%%% Startup %%%%%%%%%%%%
if measureNoise == 1
    if first 
        uref = u_ref;
        yref = y;
        first = false;
        yh = yref;
        yl = yref;
    end
    u = uref;
    if sample < noiseMeasureTime/t_sample
        yh = max(yh,y);
        yl = min(yl,y);
    else
        noise = (yh-yl)/2;
        yref = (yh+yl)/2;
        %yref = y; % Could test the latest value instead of average?
        resultvec(15) = yref;
        resultvec(16) = uref;
        h = max(2*noise, def_h);
        measureNoise = 0;
        startup = 1;
        resultvec(23) = t;
    end
elseif startup == 1
    exp_t = sample-noiseMeasureTime/t_sample;
    a = uref-c;
        u = a+c*b^(exp_t/tff);
        if u > relayMaxDev+uref
            u = relayMaxDev+uref;
        end
        if exp_t > 1
            ydev = y-yref; 
            if abs(ydev) > h % outside hysteresis, stop startup and decide Ksign
                Ksign = ydev/abs(ydev);
                if bigYup == 1
                    d1 = min(relayMaxDev, gamma*abs(u-uref));
                    d2 = d1/gamma;
                else
                    d2 = min(relayMaxDev, gamma*abs(u-uref));
                    d1 = d2/gamma;
                end
                startup = 0;
            elseif exp_t > tff
                u = uref+relayMaxDev;
            end
        end
elseif run_exp == 1
    %%%%%% Update amplitudes %%%%%%%
    u_on = uref+Ksign*d1;
    u_off = uref-Ksign*d2;
    %%%%%% Calculate new u %%%%%%%%%
    u = rel_func(y,u_old,u_on, u_off,yref,h);
else 
    u = 0; %Shouldn't be needed?
end

%%%%%%% At switching points %%%%%%%
if sample>1 && (u-uref)*(u_old-uref) < 0
    switching_times(switch_index) = t;
    if switch_index > 2
        tp = switching_times(switch_index)-switching_times(switch_index-2);
        resultvec(19) = tp;
    end
    if switch_index == 3 % Step in yref/uref after two switches
        yref = yref+ystep*h;
        uref = uref+(d1+d2)/2*Ksign*ustep;
    end
    if switch_index > maxSwitches
        done_per = 1;
        resultvec(17) = t;
    end
    switch_index = switch_index+1;
end
%%%% store data %%%%%%
u_old = u;
end

function u = rel_func(y,uold,uon,uoff,yref,h)
  if y <= yref-h
    u = uon;
  elseif y < yref+h && y > yref-h
    u = uold;
  else u = uoff;
  end
end

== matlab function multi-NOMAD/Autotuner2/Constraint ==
%function stop = Constraint(tstop, time, done)
function stop = Constraint(time, all_done, timeAfterExp)
%#codegen
persistent tstopp first
if isempty(tstopp)
    tstopp = 10000;
    first = true;
end
if all_done == 1 && first 
    tstopp = time;
    first = false;
end
if time > tstopp+timeAfterExp;
    stop = 1;
else
    stop = 0;
end

== matlab function multi-NOMAD/Autotuner2/relay_exp
 ==
function [result, u, done]= relay_exp(relay_par, e,t, u_ref, run_exp)


%%%%%%%%%% Definitions and default values %%%%%%%%%%%%%%
y = -e;
% Relay parameters, values from workspace.
persistent d1 d2 u_on u_off h
gamma = relay_par(2); % index 2 is gamma, 11 is gamma2 
t_sample = relay_par(3);
bigYup = relay_par(6);
relayMaxDev = relay_par(7);
def_h = relay_par(8);
noiseMeasureTime = relay_par(9);
maxSwitches = relay_par(12);
ystep = relay_par(13);
ustep = relay_par(14);

persistent yref uref
if isempty(d2)
    h=def_h; % these values will be re-assigned later and never used. 
    d1 = gamma;
    d2 = 1;
    u_on =  d1;
    u_off = -d2;
    uref = 0;
    yref = 0;
end

persistent u_old resultvec
if isempty(u_old)
    u_old = uref;
    resultvec = zeros(23,1);
end

persistent sample
if isempty(sample)
    sample = 0;
end

persistent startup Ksign
if isempty(Ksign)
    Ksign = 1;  % Is re-assigned during at the startup phase
end

persistent param done_per
if isempty(param)
    param = [1.1, 16, 0]; % Quadtank minfas (should be an input somehow if existing PID parameters are used to bring it to its working point)
    done_per = 0;
end
PID_param = param;
done = done_per;

% To handle switches
persistent switching_times switch_index 
if isempty(switching_times)
    switching_times = zeros(1,20);
    switch_index = 1;
end

%%%%%%%%% Startup  params %%%%%%%%%%%
persistent a b c tff exp_t yh yl measureNoise first
if isempty(startup)
    tff = 5/t_sample; % According to Tore about 3-5s is appropriate for the startup growth 
    b = 40;
    c = relayMaxDev/(b-1);
    a = uref-c;
    measureNoise = 1;
    startup = 0;
    yh = 0;
    yl = 0;
    first = true;
end
%%%%%%%%%%%%%%%%%%%%%%%%%%%%%%%%%%%%%%%%%%%%%%%

result = resultvec;
if run_exp == 0
    u = 0;
    PID_param = param;
    return
end

%%%%%%%%%%%%% Program running %%%%%%%%%%%%%%%%%
sample = sample+1;

%%%%%%%%% Startup %%%%%%%%%%%%
if measureNoise == 1
    if first 
        uref = u_ref;
        yref = y;
        first = false;
        yh = yref;
        yl = yref;
    end
    u = uref;
    if sample < noiseMeasureTime/t_sample
        yh = max(yh,y);
        yl = min(yl,y);
    else
        noise = (yh-yl)/2;
        yref = (yh+yl)/2;
        %yref = y; % Could test the latest value instead of average?
        resultvec(15) = yref;
        resultvec(16) = uref;
        h = max(2*noise, def_h);
        measureNoise = 0;
        startup = 1;
        resultvec(23) = t;
    end
elseif startup == 1
    exp_t = sample-noiseMeasureTime/t_sample;
    a = uref-c;
        u = a+c*b^(exp_t/tff);
        if u > relayMaxDev+uref
            u = relayMaxDev+uref;
        end
        if exp_t > 1
            ydev = y-yref; 
            if abs(ydev) > h % outside hysteresis, stop startup and decide Ksign
                Ksign = ydev/abs(ydev);
                if bigYup == 1
                    d1 = min(relayMaxDev, gamma*abs(u-uref));
                    d2 = d1/gamma;
                else
                    d2 = min(relayMaxDev, gamma*abs(u-uref));
                    d1 = d2/gamma;
                end
                startup = 0;
            elseif exp_t > tff
                u = uref+relayMaxDev;
            end
        end
elseif run_exp == 1
    %%%%%% Update amplitudes %%%%%%%
    u_on = uref+Ksign*d1;
    u_off = uref-Ksign*d2;
    %%%%%% Calculate new u %%%%%%%%%
    u = rel_func(y,u_old,u_on, u_off,yref,h);
else 
    u = 0; % Shouldn't be needed?
end

%%%%%%% At switching points %%%%%%%
if sample>1 && (u-uref)*(u_old-uref) < 0
    switching_times(switch_index) = t;
    if switch_index > 2
        tp = switching_times(switch_index)-switching_times(switch_index-2);
        resultvec(19) = tp;
    end
    if switch_index == 3 % Step in yref/uref after two switches
        yref = yref+ystep*h;
        uref = uref+(d1+d2)/2*Ksign*ustep;
    end
    if switch_index > maxSwitches
        done_per = 1;
        resultvec(17) = t;
    end
    switch_index = switch_index+1;
end
%%%% store data %%%%%%
u_old = u;
end

function u = rel_func(y,uold,uon,uoff,yref,h)
  if y <= yref-h
    u = uon;
  elseif y < yref+h && y > yref-h
    u = uold;
  else u = uoff;
  end
end
